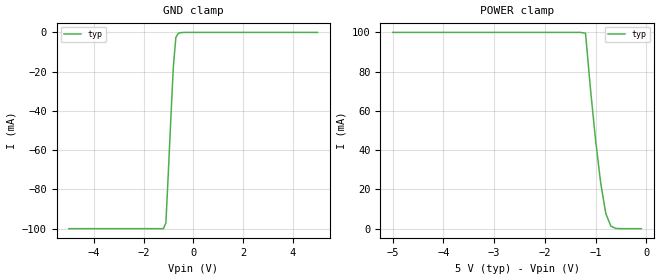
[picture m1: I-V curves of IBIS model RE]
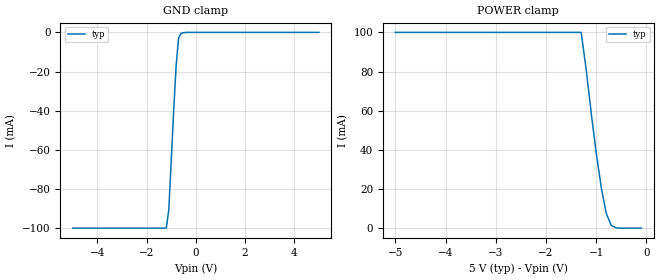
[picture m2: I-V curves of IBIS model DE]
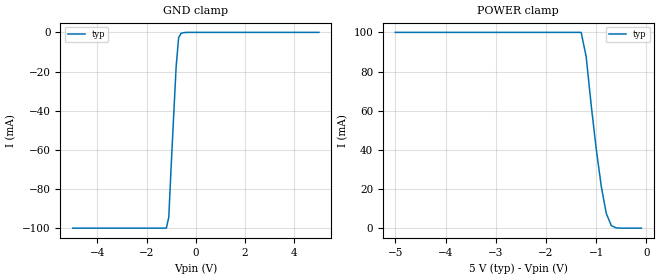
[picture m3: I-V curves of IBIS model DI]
| IBIS file 485.ibs created at Maxim Integrated Products
[IBIS ver]   2.1
[File name]   485.ibs
[File Rev]   1.0
[Date]   December 05, 2002
[Source]   Rise and fall ramps, and IV curves were taken on the bench
   using an Oscilloscope and Semiconductor Parameter Analyzer.
[Notes]   This is a Low-Power Slew-Rate-Limited RS422 Transceiver.
[Disclaimer] Maxim Integrated Products hereby grants the user of this
   IBIS model a non-exclusive, nontransferable license to
   use this IBIS model under the following terms. Before
   using this IBIS model, the user should read this license.
   If the user does not accept these terms, the IBIS model
   should be returned to Maxim Integrated Products within 30
   days. The user is granted this license only to use the
   IBIS model and is not granted rights to sell, load, rent,
   lease or license the IBIS model in whole or in part, or
   in modified form to anyone other than user. User may modify
   the IBIS model to suit its specific applications but rights
   to derivative works and such modifications shall belong to
   Maxim Integrated Products. This IBIS model is provided on
   an "AS IS" basis and Maxim Integrated Products makes
   absolutely no warranty with respect to the information
   contained herein. MAXIM INTEGRATED PRODUCTS DISCLAIMS AND
   CUSTOMER WAIVES ALL WARRANTIES, EXPRESS OR IMPLIED,
   INCLUDING WARRANTIES OF MERCHANTABILITY OR FITNESS FOR A
   PARTICULAR PURPOSE. The entire risk as to quality and
   performance is with the Customer. ACCORDINGLY, IN NO EVENT
   SHALL THE COMPANY BE LIABLE FOR ANY DAMAGES, WHETHER IN
   CONTRACT OR TORT, INCLUDING ANY LOST PROFITS OR OTHER
   INCIDENTAL, CONSEQUENTIAL, EXEMPLARY, OR PUNITIVE DAMAGES
   ARISING OUT OF THE USE OR APPLICATION OF THE IBIS model
   provided in this package.Further, Maxim Integrated Products
   reserves the right to make changes without notice to any
   product herein to improve reliability, function, or design.
   Maxim Integrated Products does not convey any license under
   patent rights or any other intellectual property rights,
   including those of third parties. Maxim Integrated Products
   is not obligated to provide maintenance or support for the
   licensed IBIS model.
[Copyright]   COPYRIGHT MAXIM INTEGRATED PRODUCTS 2002 ALL RIGHTS PRESERVE.
|   Component MAX485
[Component]   MAX485
[Manufacturer]   Maxim Integrated Products
[Package]
| variable   typ   min   max
R_pkg   55.5m   NA   NA
L_pkg   1.57nH   NA   NA
C_pkg   0.252pF   NA   NA
[Pin]  signal_name   model_name   R_pin   L_pin   C_pin
1   RO   RO
2   REB   RE
3   DE   DE
4   DI   DI
5   GND   GND
6   A   Driver_IO
7   B   Driver_IO
8   VCC   POWER
| Models and submodels in the file (5): RE (Input), DE (Input), DI (Input), RO (3-state), Driver_IO (I/O)
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|   Driver Output Receiver Enable
[Model]   RE
|Signals   REB
Model_type   Input
Enable   Active-Low
Vinl = 0.8V
Vinh = 2.0V
C_comp   0.538pF   NA   NA
[Temperature Range]   25   -40   85
[Voltage Range]   5.00V   4.75V   5.25V
[POWER Clamp Reference]   5.00V   4.75V   5.25V
[GND Clamp Reference]   0.00V   0.00V   0.00V
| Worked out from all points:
|   GND clamp passes 1 mA (typ) near -0.63 V on its own axis
|   POWER clamp passes 1 mA (typ) near -0.68 V on its own axis
[POWER_clamp]
| Note that the[POWER_clamp]voltage table is referenced to Vcc
| and is calculated using Vtable=Vcc - Vmeasured.
| Also, the Semiconductor Parameter Analyzer (Force and Sense)
| clamps the supply current to 100mA to protect the system.
| V(V)  I(typ)   I(min)  I(max)
-5V       100mA      NA         NA
-1.3V     100mA      NA         NA
-1.2V     99.59mA    NA         NA
-1.1V     70.58mA    NA         NA
-1V       44.72mA    NA         NA
-900mV    23.15mA    NA         NA
-800mV    7.748mA    NA         NA
-700mV    1.253mA    NA         NA
-600mV    91.95uA    NA         NA
-100mV    0A         NA         NA
[GND_clamp]
| Note that the[GND_clamp]voltage table is referenced to Gnd.
| Also, the Semiconductor Parameter Analyzer (Force and Sense)
| clamps the supply current to 100mA to protect the system.
| V(V)  I(typ)   I(min)  I(max)
-5V       -100mA     NA         NA
-1.2V     -100mA     NA         NA
-1.1V     -96.97mA   NA         NA
-1V       -70.59mA   NA         NA
-900mV    -43.26mA   NA         NA
-800mV    -17.31mA   NA         NA
-700mV    -2.579mA   NA         NA
-600mV    -464.4uA   NA         NA
-300mV    -1.684uA   NA         NA
5V        0A         NA         NA
|   Driver Output Transmitter Enable
[Model]   DE
|Signals   DE
Model_type   Input
Enable   Active-High
Vinl = 0.8V
Vinh = 2.0V
C_comp   0.538pF   NA   NA
[Temperature Range]   25   -40   85
[Voltage Range]   5.00V   4.75V   5.25V
[POWER Clamp Reference]   5.00V   4.75V   5.25V
[GND Clamp Reference]   0.00V   0.00V   0.00V
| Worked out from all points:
|   GND clamp passes 1 mA (typ) near -0.62 V on its own axis
|   POWER clamp passes 1 mA (typ) near -0.67 V on its own axis
[POWER_clamp]
| Note that the[POWER_clamp]voltage table is referenced to Vcc
| and is calculated using Vtable=Vcc - Vmeasured.
| Also, the Semiconductor Parameter Analyzer (Force and Sense)
| clamps the supply current to 100mA to protect the system.
| V(V)  I(typ)   I(min)  I(max)
-5V       100mA      NA         NA
-1.3V     100mA      NA         NA
-1.2V     81.06mA    NA         NA
-1.1V     58.85mA    NA         NA
-1V       38.47mA    NA         NA
-900mV    20.82mA    NA         NA
-800mV    7.529mA    NA         NA
-700mV    1.353mA    NA         NA
-600mV    108.3uA    NA         NA
-100mV    0A         NA         NA
[GND_clamp]
| Note that the[GND_clamp]voltage table is referenced to Gnd.
| Also, the Semiconductor Parameter Analyzer (Force and Sense)
| clamps the supply current to 100mA to protect the system.
| V(V)  I(typ)   I(min)  I(max)
-5V       -100mA     NA         NA
-1.2V     -100mA     NA         NA
-1.1V     -90.71mA   NA         NA
-1V       -65.73mA   NA         NA
-900mV    -39.73mA   NA         NA
-800mV    -16.86mA   NA         NA
-700mV    -2.904mA   NA         NA
-600mV    -495.1uA   NA         NA
-300mV    -2.087uA   NA         NA
5V        0A         NA         NA
|   Driver Transmitter Input
[Model]   DI
|Signals   DI
Model_type   Input
Enable   Active-High
Vinl = 0.8V
Vinh = 2.0V
C_comp   0.538pF   NA   NA
[Temperature Range]   25   -40   85
[Voltage Range]   5.00V   4.75V   5.25V
[POWER Clamp Reference]   5.00V   4.75V   5.25V
[GND Clamp Reference]   0.00V   0.00V   0.00V
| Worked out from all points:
|   GND clamp passes 1 mA (typ) near -0.62 V on its own axis
|   POWER clamp passes 1 mA (typ) near -0.68 V on its own axis
[POWER_clamp]
| Note that the[POWER_clamp]voltage table is referenced to Vcc
| and is calculated using Vtable=Vcc - Vmeasured.
| Also, the Semiconductor Parameter Analyzer (Force and Sense)
| clamps the supply current to 100mA to protect the system.
| V(V)  I(typ)   I(min)  I(max)
-5V       100mA      NA         NA
-1.3V     100mA      NA         NA
-1.2V     87.55mA    NA         NA
-1.1V     62.84mA    NA         NA
-1V       40.47mA    NA         NA
-900mV    21.45mA    NA         NA
-800mV    7.513mA    NA         NA
-700mV    1.287mA    NA         NA
-600mV    97.96uA    NA         NA
-100mV    0A         NA         NA
[GND_clamp]
| Note that the[GND_clamp]voltage table is referenced to Gnd.
| Also, the Semiconductor Parameter Analyzer (Force and Sense)
| clamps the supply current to 100mA to protect the system.
| V(V)  I(typ)   I(min)  I(max)
-5V       -100mA     NA         NA
-1.2V     -100mA     NA         NA
-1.1V     -94.53mA   NA         NA
-1V       -67.6mA    NA         NA
-800mV    -17.49mA   NA         NA
-700mV    -2.703mA   NA         NA
-600mV    -475.3uA   NA         NA
-300mV    -1.824uA   NA         NA
5V        0A         NA         NA
